//05.04.99
//Umstrukturierung, Aufruf FB2 mit Multiinstanz-DB
//Lesen von numMagPlaceParam bei Neustart da Änderung Anzahl Par. in SW 5 (8)
//DB97 und DB98 entfallen da Aufruf FB2 mit Multiiinstanz-DB
//neue Fkt: TNr_write=1, Vorgabe TNummer in TNr von extern
//

FUNCTION_BLOCK FB 92
TITLE = GET_LOC
VERSION : 2.0

VAR_INPUT
    Req: Bool; // Start Zustände lesen
    GetWkz: Bool; // Werkzeugzustand lesen
    MagNr: Int; // Magazin-Nr. Daten lesen
    LocNr: Int; // Platz-Nr. Daten lesen
END_VAR

VAR_OUTPUT
    NDR: Bool; // Leerplatz gefunden
    Error: Bool; // Fehler
    State: Word; // Fehler-Nummer
END_VAR

VAR
    TOANr: Byte:=b#16#1; // TOA-Bereich
    TNr_write: Bool:=False; // T-Nummer von Anwender versorgt
    numMagPlaceParams: Word; // Anzahl Parameter eines Magzinplatzes
    numPlacePar_read: Bool; //Variable nummagplaceparams lesen nach Neustart
    numPlacePar_Error: Bool; // Fehler bei Variable nummagplaceparams lesen
    numPlacePar_ok: Bool; // Variable numMagPlaceParams gelesen ohne Fehler
    Activ: Bool; // Baustein aktiv
    Schrittregister : BYTE ;
    StateFB2_Gesp: Word; // Ausgang State FB2 T-Nr. lesen gespeichert
    Reserve: ARRAY  [0 .. 4 ] OF Int;
    TNr: 	Int; // logische T-Nummer
    Loc_Zu:	Int; // Platzzustand
    Groesse_links: Int; // Größe nach links in Halbplätzen
    Groesse_rechts: Int; // Größe nach rechts in Halbplätzen
    Groesse_oben: Int; // Größe nach oben in Halbplätzen
    Groesse_unten: Int; // Größe nach unten in Halbplätzen
    WZTyp:	Int; // Magazinplatztyp
    WZStatus:	Int; // Werkzeugstatus
    GET_FB2 : FB 2;
END_VAR

VAR_TEMP
    Error_FB2: Bool; // Error FB2
    NDR_FB2: Bool; // Auftrag beendet FB2
    LocLine1: Word; // Zeilenadresse Addr1
    LocLine2: Word; // Zeilenadresse Addr2
    Column_FB2: Word; // Spaltenadresse FB2
    State_FB2: Word; // Fehler-Nr. FB2
END_VAR

Begin
     UN   DB8.DBX45.0;
     SPB  ANF1;		// Neustart ? Nein ->
     CALL #GET_FB2 (
     Req:= FALSE);
     SET;
     R    numPlacePar_Error;
     S    numPlacePar_read;
     R    numPlacePar_ok;
     SPA  LOEP;
ANF1:UN   numPlacePar_read;
     SPB  ANF2;
     call #GET_FB2 ( // -- Anzahl Parameter eines Magazinplatz lesen --
     Req:=TRUE, // Variable lesen
     NumVar:= 1, // Anzahl der zu lesenden Variablen
     Addr1:=WZV_VAR.N_Y_numMagPlaceParams_27, // Variable numMagPlaceParams
     Error:=#Error_FB2, // NC_VAR lesen beendet mit Fehler
     NDR:=#NDR_FB2, // NC_VAR lesen beendet ohne Fehler
     State:=#State_FB2, // Fehler-Nummer bei Error = 1
     RD1:=numMagPlaceParams); // Wert in numMagPlaceParams
     UN    #NDR_FB2; // Lesen beendet ohne Fehler
     UN    #Error_FB2; // Lesen beendet mit Fehler
     SPB   ENDE; // Lesen beendet ? Nein ->
     call #GET_FB2 ( // FB2 freigeben
     Req:=False);
     UN    #Error_FB2;
     R     numPlacePar_read;
     S     numPlacePar_ok;
     SPB   ENDE; // Lesen beendet mit Fehler ? Nein ->
     L     6;
     L     #State_FB2;
     ==I;
     SPB   ENDE; // FIFO voll -> Lesen wiederholen
     S     numPlacePar_Error;
     R     numPlacePar_read;
     T     StateFB2_Gesp; // Fehlernummer speichern
     SPA   ENDE;
ANF2:U   Req;
     SPB ANF;
LOEP:R    NDR; // Ausgangsparameter Done nur 1 PLC-Zyklus
     R    Error; // Ausgangsparameter Error nur 1 PLC-Zyklus
     R    Activ;
     L    0;
     T    State; // Fehler-Nr. = 0
     SPA  ENDE;
ANF: U    Activ;
     SPB  SPRG; // Baustein aktiv ? Ja ->
     U   numPlacePar_Error;
     ON  numPlacePar_ok;
     L	7;
     SPB  FEHL; // Fehler bei Variable numMagPlaceParams lesen ->
     S    Activ; // Hilfsvariable vorbesetzen
     R    NDR;
     R    Error;
     L    0;
     T    State; // Fehler-Nr. = 0
     U    TNr_write;
     U    GetWkz;
     SPB  QFEH; // T-Nr. von Anwender ? ->
     T    Schrittregister;
SPRG:L    Schrittregister;
     SPL  FEHS; // Sprungverteiler
     SPA  SR1; // Magazinplatzdaten lesen
     SPA  SR2; // WZ-Daten lesen
FEHS:L 6;
     SPA  FEHL;
SR1: L    MagNr; // ----Schritt 1: T-Nr. lesen --------------------
     T    Column_FB2; // Spalte Addr1 = Magazin-Nummer
     L    LocNr; // Platz-Nr. Zwischenspeicher
     +    -1;
     L    numMagPlaceParams; // Anzahl Parameter pro MagPlatz
     *I; // (PlatzNr.-1)*numMagPlaceParams+Parameter-Nr.
     +    3;
     T    #LocLine1; // Zeile Addr1 = T-Nr.
     +    2;
     T    #LocLine2; // Zeile Addr2 = Platzzustand
     call #GET_FB2 ( // -- Magazinplatzdaten lesen --
     Req:=TRUE, // Variable lesen
     NumVar:= 2, // Anzahl der zu lesenden Variablen
     Addr1:=WZV_VAR.T0_TP_placeData0_0, // T-Nummer von WZ in Zwischenspeicher
     Unit1:=TOANr, // Bereich = TOA 1
     Column1:=#Column_FB2, // Spaltenadresse
     Line1:=#LocLine1, // Zeilenadresse
     Addr2:=WZV_VAR.T0_TP_placeData0_0, // T-Nummer von WZ in Zwischenspeicher
     Unit2:=TOANr, // Bereich = TOA 1
     Column2:=#Column_FB2, // Spaltenadresse
     Line2:=#LocLine2, // Zeilenadresse
     Error:=#Error_FB2, // NC_VAR lesen beendet mit Fehler
     NDR:=#NDR_FB2, // NC_VAR lesen beendet ohne Fehler
     State:=#State_FB2, // Fehler-Nummer bei Error = 1
     RD1:=TNr, // Zielbereich für T-Nummer
     RD2:=Loc_Zu); // Zielbereich für Platzzustand
     UN    #NDR_FB2; // Lesen beendet ohne Fehler
     UN    #Error_FB2; // Lesen beendet mit Fehler
     SPB   ENDE; // Lesen beendet ? Nein ->
     call #GET_FB2 ( // FB2 freigeben
     Req:=False);
     UN    #Error_FB2;
     SPB   QFEH; // Lesen beendet mit Fehler ? Nein ->
     L     6;
     L     #State_FB2;
     ==I;
     SPB   ENDE;
     T     StateFB2_Gesp; // Fehlernummer speichern
     L     1; // Fehler-Nummer FB 91 = 1
     SPA   FEHL;
QFEH:UN    GetWkz;
     SPB   DONE; // Nur Platzzustand lesen ? ->
     L     TNr;	// logische T-Nummer von WZ in Zwischenspeicher
     L     0;
     ==I;
     L     2;
     SPB   FEHL; // T-Nr. in Zwischensp. = 0 ? -> Fehler
     L     1;
     T     Schrittregister;
SR2: L     TNr; // logische T-Nr. = Zeilenadresse
     T    #LocLine1; // Zeile Addr = T-Nr.
FB2: call #GET_FB2( // -- Werkzeugdaten lesen --
     Req:=TRUE,
     NumVar:= 6,
     Addr1:=WZV_VAR.T0_TD_toolState0_0, // Größe nach links in Halbplätze
     Unit1:=TOANr, // Bereich = TOA 1
     Column1:=w#16#0003, // Spaltenadresse
     Line1:=#LocLine1, // Zeilenadresse
     Addr2:=WZV_VAR.T0_TD_toolState0_0, // Größe nach rechts in Halbplätze
     Unit2:=TOANr, // Bereich = TOA 1
     Column2:=w#16#0004, // Spaltenadresse
     Line2:=#LocLine1, // Zeilenadresse
     Addr3:=WZV_VAR.T0_TD_toolState0_0, // Größe nach oben in Halbplätze
     Unit3:=TOANr, // Bereich = TOA 1
     Column3:=w#16#0005, // Spaltenadresse
     Line3:=#LocLine1, // Zeilenadresse
     Addr4:=WZV_VAR.T0_TD_toolState0_0, // Größe nach unten in Halbplätze
     Unit4:=TOANr, // Bereich = TOA 1
     Column4:=w#16#0006, // Spaltenadresse
     Line4:=#LocLine1, // Zeilenadresse
     Addr5:=WZV_VAR.T0_TD_toolState0_0, // Magazinplatztyp
     Unit5:=TOANr, // Bereich = TOA 1
     Column5:=w#16#0007, // Spaltenadresse
     Line5:=#LocLine1, // Zeilenadresse
     Addr6:=WZV_VAR.T0_TD_toolState0_0, // WZ-Status
     Unit6:=TOANr, // Bereich = TOA 1
     Column6:=w#16#0008, // Spaltenadresse
     Line6:=#LocLine1, // Zeilenadresse
     Error:=#Error_FB2, // NC_VAR lesen beendet mit Fehler
     NDR:=#NDR_FB2, // NC_VAR lesen beendet ohne Fehler
     State:=#State_FB2, // Fehler-Nummer bei Error = 1
     RD1:=Groesse_links, // Größe nach links in Halbplätze
     RD2:=Groesse_rechts, // Größe nach rechts in Halbplätze
     RD3:=Groesse_oben, // Größe nach oben in Halbplätze
     RD4:=Groesse_unten, // Größe nach unten in Halbplätze
     RD5:=WZTyp, // Magazinplatztyp
     RD6:=WZStatus); // WZ-Status
     UN    #NDR_FB2; // Lesen beendet ohne Fehler
     UN    #Error_FB2; // Lesen beendet mit Fehler
     SPB   ENDE; // Lesen beendet ? Nein ->
     call #GET_FB2 ( // FB2 freigeben
     Req:=False);
     UN    #Error_FB2;
     SPB   DONE; // Lesen beendet mit Fehler ? Nein ->
     L	6;
     L	#State_FB2;
     ==I;
     SPB	ENDE;
     T StateFB2_Gesp; // Fehlernummer speichern
     L     3; // Fehler-Nummer FB 92 = 3
     SPA   FEHL;
DONE:S     NDR;
     SPA   SR0;
FEHL:T     State; // Fehler-Nummer FB92 ausgeben
     S     Error;
SR0: R     Activ;
     L     0;
     T     Schrittregister; // Schrittregister auf Anfang
ENDE:NOP   0
END_FUNCTION_BLOCK

DATA_BLOCK db 92

        VERSION: 2.0

fb 92
Begin
END_DATA_BLOCK

